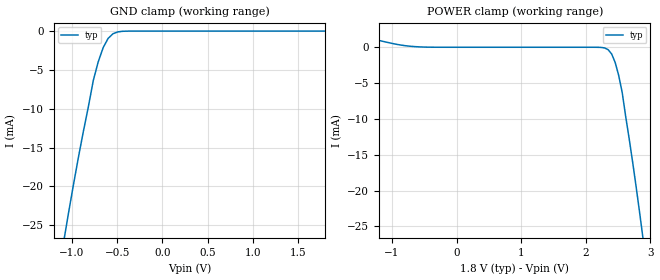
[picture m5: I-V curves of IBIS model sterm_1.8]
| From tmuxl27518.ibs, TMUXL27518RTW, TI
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| sterm_1.8
[Model]   sterm_1.8
Model_type   Terminator
|   typ   min   max
C_comp   4.014581e-12   NA   NA
[Voltage Range]   1.8   NA   NA
[Temperature Range]   27   NA   NA
[Power Clamp Reference]   1.8   NA   NA
[GND Clamp Reference]   0   NA   NA
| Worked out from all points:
|   GND clamp passes 1 mA (typ) near -0.60 V on its own axis
|   POWER clamp passes 1 mA (typ) near -1.22 V on its own axis
[GND Clamp]
|   Voltage   I(typ)   I(min)   I(max)
-3.6V     -265.3mA   NA         NA
-1.091V   -27.09mA   NA         NA
-1.036V   -23.33mA   NA         NA
-927.3mV  -16.19mA   NA         NA
-763.6mV  -6.356mA   NA         NA
-709.1mV  -3.951mA   NA         NA
-654.5mV  -2.128mA   NA         NA
-600mV    -944.6uA   NA         NA
-545.5mV  -336.9uA   NA         NA
-490.9mV  -99.04uA   NA         NA
-381.8mV  -5.247uA   NA         NA
1.8V      283.7pA    NA         NA
[POWER Clamp]
|   Voltage   I(typ)   I(min)   I(max)
-1.8V     2.344mA    NA         NA
-654.5mV  94.12uA    NA         NA
2.182V    -5.247uA   NA         NA
2.345V    -336.9uA   NA         NA
2.4V      -944.6uA   NA         NA
2.455V    -2.128mA   NA         NA
2.509V    -3.951mA   NA         NA
2.564V    -6.356mA   NA         NA
2.727V    -16.19mA   NA         NA
2.836V    -23.33mA   NA         NA
2.891V    -27.09mA   NA         NA
3.6V      -82.13mA   NA         NA
